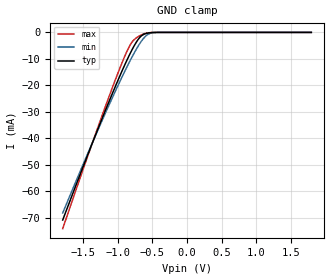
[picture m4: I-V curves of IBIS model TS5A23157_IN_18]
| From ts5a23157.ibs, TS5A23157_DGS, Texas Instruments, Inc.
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[Model]   TS5A23157_IN_18
Model_type  Input
Vinl=0.4875
Vinh=1.2375
| variable   typ   min   max
C_comp   2.68pF   2.18pF   3.22pF
[Temperature Range]   40   100   -40
| Ambient temperature   25   85   -40
[Voltage range]   1.8   1.65   1.95
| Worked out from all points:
|   GND clamp passes 1 mA (typ) near -0.64 V on its own axis
[GND Clamp]
| TS5A23157_IN_18
|   Voltage   I(typ)   I(min)   I(max)
-1.8V     -70.95mA   -68.28mA   -74.2mA
-1.35V    -40.46mA   -40.51mA   -40.26mA
-1.03V    -19.95mA   -21.8mA    -17.38mA
-925mV    -13.66mA   -15.99mA   -10.47mA
-850mV    -9.408mA   -12.02mA   -6.088mA
-800mV    -6.767mA   -9.489mA   -3.814mA
-745mV    -4.16mA    -6.858mA   -2.298mA
-675mV    -1.673mA   -3.868mA   -1.137mA
-605mV    -517.4uA   -1.575mA   -393.5uA
-550mV    -185.6uA   -539uA     -116.2uA
-485mV    -43.93uA   -106.4uA   -18.16uA
1.8V      41.95pA    147.4pA    23.47pA
